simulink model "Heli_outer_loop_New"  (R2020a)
settings: Solver=FixedStepDiscrete  StartTime=0.0  StopTime=10.0  FixedStep=0.01  RelTol=1e-3  EnableMultiTasking=on
model workspace (MAT data in the model file):
  Ts : Simulink.Parameter (value not decoded)
symbols that are objects in the model workspace (value not decoded): Ts
undefined symbols (not defined in the file or in its folder): DiscIntNeverNeededParam
libraries: simulink x1

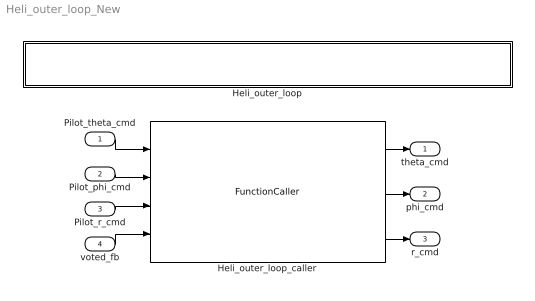
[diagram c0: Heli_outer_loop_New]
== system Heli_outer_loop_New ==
  Pilot_theta_cmd : Inport  OutMin=-32768  OutMax=32767  OutDataTypeStr=int16  PortDimensions=1  SampleTime=0.01
  Pilot_phi_cmd : Inport  Port=2  OutMin=-32768  OutMax=32767  OutDataTypeStr=int16  PortDimensions=1  SampleTime=0.01
  Pilot_r_cmd : Inport  Port=3  OutMin=-32768  OutMax=32767  OutDataTypeStr=int16  PortDimensions=1  SampleTime=0.01
  voted_fb : Inport  Port=4  OutMin=-180  OutMax=180  OutDataTypeStr=double  PortDimensions=5  SampleTime=0.01
  Heli_outer_loop : Subsystem  TreatAsAtomicUnit=on
  Heli_outer_loop_caller : FunctionCaller  FunctionPrototype=[theta_cmd,phi_cmd,r_cmd] = Heli_outer_loop(Pilot_theta_cmd,Pilot_phi_cmd,Pilot_r_cmd,voted_fb)
  theta_cmd : Outport  OutMin=-30  OutMax=30  OutDataTypeStr=double  PortDimensions=1  SampleTime=0.01  VectorParamsAs1DForOutWhenUnconnected=off
  phi_cmd : Outport  Port=2  OutMin=-30  OutMax=30  OutDataTypeStr=double  PortDimensions=1  SampleTime=0.01  VectorParamsAs1DForOutWhenUnconnected=off
  r_cmd : Outport  Port=3  OutMin=-30  OutMax=30  OutDataTypeStr=double  PortDimensions=1  SampleTime=0.01  VectorParamsAs1DForOutWhenUnconnected=off
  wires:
  Pilot_theta_cmd/1 -> Heli_outer_loop_caller/1
  Pilot_phi_cmd/1 -> Heli_outer_loop_caller/2
  Pilot_r_cmd/1 -> Heli_outer_loop_caller/3
  voted_fb/1 -> Heli_outer_loop_caller/4
  Heli_outer_loop_caller/1 -> theta_cmd/1
  Heli_outer_loop_caller/2 -> phi_cmd/1
  Heli_outer_loop_caller/3 -> r_cmd/1

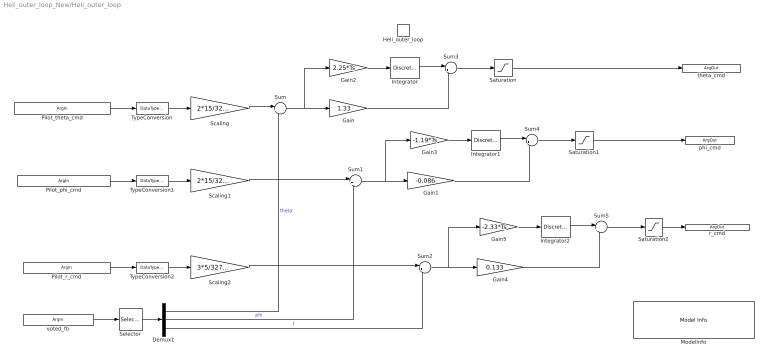
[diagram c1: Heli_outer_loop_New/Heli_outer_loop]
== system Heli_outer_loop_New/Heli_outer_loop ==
  Heli_outer_loop : TriggerPort  TriggerType=function-call  IsSimulinkFunction=on  FunctionName=Heli_outer_loop  FunctionVisibility=scoped  VariantControl=Variant  PortDimensions=1
  Demux1 : Demux  Outputs=3
  Gain : Gain  Gain=1.33
  Gain1 : Gain  Gain=-0.086
  Gain2 : Gain  Gain=2.25*Ts
  Gain3 : Gain  Gain=-1.19*Ts
  Gain4 : Gain  Gain=0.133
  Gain5 : Gain  Gain=-2.33*Ts
  Integrator : DiscreteIntegrator  IntegratorMethod=Accumulation: Forward Euler  SampleTime=-1  LimitOutput=on  UpperSaturationLimit=10  LowerSaturationLimit=-10  ICPrevOutput=DiscIntNeverNeededParam  ICPrevScaledInput=DiscIntNeverNeededParam
  Integrator1 : DiscreteIntegrator  IntegratorMethod=Accumulation: Forward Euler  SampleTime=-1  LimitOutput=on  UpperSaturationLimit=10  LowerSaturationLimit=-10  ICPrevOutput=DiscIntNeverNeededParam  ICPrevScaledInput=DiscIntNeverNeededParam
  Integrator2 : DiscreteIntegrator  IntegratorMethod=Accumulation: Forward Euler  SampleTime=-1  LimitOutput=on  UpperSaturationLimit=10  LowerSaturationLimit=-10  ICPrevOutput=DiscIntNeverNeededParam  ICPrevScaledInput=DiscIntNeverNeededParam
  ModelInfo : simulink/Model-Wide Utilities/Model Info  Frame=on  DisplayStringWithTags=|  HorizontalTextAlignment=Center  LeftAlignmentValue=0.5
      | Model Name: %<ModelName>
      | Model Version: %<ModelVersion>
      | Last Modified: %<LastModificationDate>
      | 
      | Copyright 2016 The MathWorks, Inc.
  Saturation : Saturate  UpperLimit=30  LowerLimit=-30
  Saturation1 : Saturate  UpperLimit=30  LowerLimit=-30
  Saturation2 : Saturate  UpperLimit=30  LowerLimit=-30
  Scaling : Gain  Gain=2*15/32767
  Scaling1 : Gain  Gain=2*15/32767
  Scaling2 : Gain  Gain=3*5/32767
  Selector : Selector  InputPortWidth=5  IndexOptions=Index vector (dialog)  Indices=[1 2 3]  OutputSizes=1
  Sum : Sum  Inputs=|+-  InputSameDT=on
  Sum1 : Sum  Inputs=|+-  InputSameDT=on
  Sum2 : Sum  Inputs=|+-  InputSameDT=on
  Sum3 : Sum  Inputs=|++
  Sum4 : Sum  Inputs=|++
  Sum5 : Sum  Inputs=|++
  TypeConversion : DataTypeConversion  OutDataTypeStr=double
  TypeConversion1 : DataTypeConversion  OutDataTypeStr=double
  TypeConversion2 : DataTypeConversion  OutDataTypeStr=double
  Pilot_theta_cmd : ArgIn  OutMin=-32768  OutMax=32767  OutDataTypeStr=int16  ArgumentName=Pilot_theta_cmd
  Pilot_phi_cmd : ArgIn  Port=2  OutMin=-32768  OutMax=32767  OutDataTypeStr=int16  ArgumentName=Pilot_phi_cmd
  Pilot_r_cmd : ArgIn  Port=3  OutMin=-32768  OutMax=32767  OutDataTypeStr=int16  ArgumentName=Pilot_r_cmd
  voted_fb : ArgIn  Port=4  OutMin=-180  OutMax=180  PortDimensions=5  ArgumentName=voted_fb
  theta_cmd : ArgOut  OutMin=-30  OutMax=30  ArgumentName=theta_cmd
  phi_cmd : ArgOut  Port=2  OutMin=-30  OutMax=30  ArgumentName=phi_cmd
  r_cmd : ArgOut  Port=3  OutMin=-30  OutMax=30  ArgumentName=r_cmd
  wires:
  Selector/1 -> Demux1/1
  Scaling2/1 -> Sum2/1
  Scaling1/1 -> Sum1/1
  Saturation/1 -> theta_cmd/1
  TypeConversion2/1 -> Scaling2/1
  Pilot_r_cmd/1 -> TypeConversion2/1
  Sum2/1 -> Gain5/1, Gain4/1
  Gain3/1 -> Integrator1/1
  Integrator/1 -> Sum3/1
  Demux1/3 -> Sum2/2  "r"
  Scaling/1 -> Sum/1
  Pilot_phi_cmd/1 -> TypeConversion1/1
  Demux1/2 -> Sum1/2  "phi"
  Gain2/1 -> Integrator/1
  Sum3/1 -> Saturation/1
  Saturation1/1 -> phi_cmd/1
  TypeConversion1/1 -> Scaling1/1
  Gain/1 -> Sum3/2
  Gain5/1 -> Integrator2/1
  Pilot_theta_cmd/1 -> TypeConversion/1
  Integrator1/1 -> Sum4/1
  Sum4/1 -> Saturation1/1
  Gain1/1 -> Sum4/2
  Integrator2/1 -> Sum5/1
  Sum/1 -> Gain/1, Gain2/1
  Demux1/1 -> Sum/2  "theta"
  Gain4/1 -> Sum5/2
  Sum1/1 -> Gain3/1, Gain1/1
  Sum5/1 -> Saturation2/1
  Saturation2/1 -> r_cmd/1
  TypeConversion/1 -> Scaling/1
  voted_fb/1 -> Selector/1
